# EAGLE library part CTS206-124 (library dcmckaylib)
DIP Switch 4 Position SPDT CTS
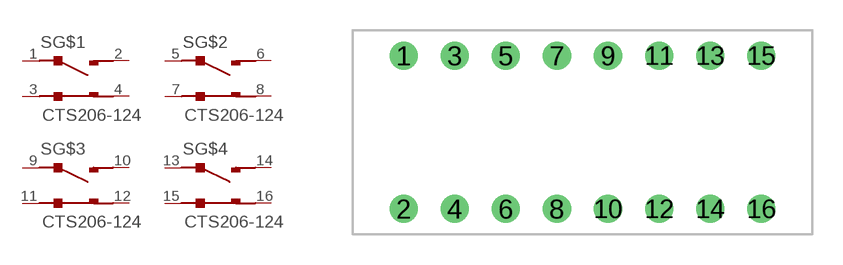
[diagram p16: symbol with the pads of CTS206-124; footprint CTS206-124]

Designator prefix S; gates G$1=SPDTSWITCH2 G$2=SPDTSWITCH2 G$3=SPDTSWITCH2 G$4=SPDTSWITCH2

## CTS206-124  [CTS206-124]
1  G$1:P$1
2  G$1:P$2
3  G$1:P$3
4  G$1:P$4
5  G$2:P$1
6  G$2:P$2
7  G$2:P$3
8  G$2:P$4
9  G$3:P$1
10  G$3:P$2
11  G$3:P$3
12  G$3:P$4
13  G$4:P$1
14  G$4:P$2
15  G$4:P$3
16  G$4:P$4

## Footprint CTS206-124 (pad centres in mm)
drill 0.889: 1 -10.16,3.81; 2 -10.16,-3.81; 3 -7.62,3.81; 4 -7.62,-3.81; 5 -5.08,3.81; 6 -5.08,-3.81; 7 -2.54,3.81; 8 -2.54,-3.81; 9 0,3.81; 10 0,-3.81; 11 2.54,3.81; 12 2.54,-3.81; 13 5.08,3.81; 14 5.08,-3.81; 15 7.62,3.81; 16 7.62,-3.81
